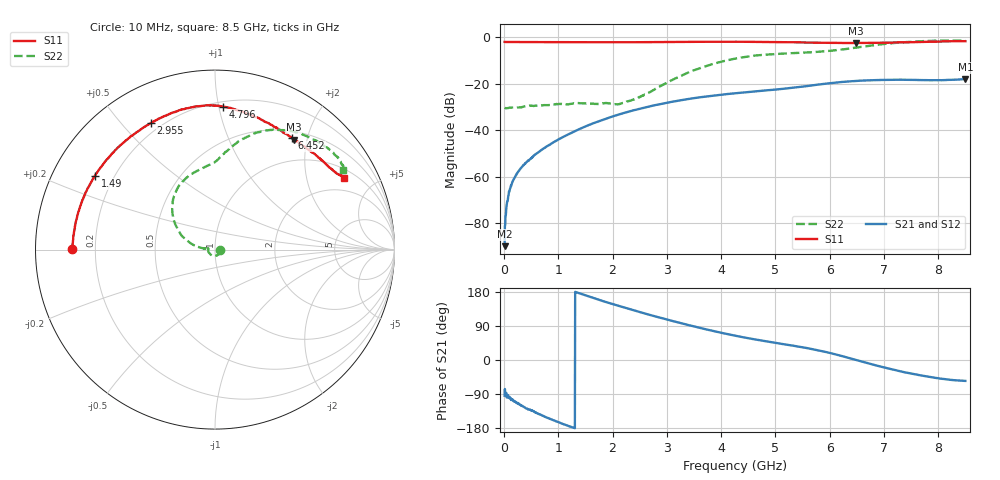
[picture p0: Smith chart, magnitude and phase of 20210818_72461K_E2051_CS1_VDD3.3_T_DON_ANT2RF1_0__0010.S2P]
!Agilent Technologies,E5071C,MY46417908,A.11.23
!Date: Wed Aug 18 14:23:20 2021
!Data & Calibration Information:
!Freq	S11:SOLT2(ON)	S21:SOLT2(ON)	S12:SOLT2(ON)	S22:SOLT2(ON)
!PortZ  Port1:50+j0  Port2:50+j0
!Above PortZ is port z conversion or system Z0 setting when saving the data.
!When reading, reference impedance value at option line is always used.
# Hz S dB R 50
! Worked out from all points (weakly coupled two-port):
!   1601 points, 10 MHz to 8.5 GHz, reference 50 ohm
!   highest |S21| = -17.98 dB at 8.5 GHz (marker M1); lowest = -89.8 dB at 10 MHz (marker M2)
!   lowest |S11| = -2.5 dB at 6.489 GHz (marker M3), VSWR 7.12, Z = 31.3 + j88.8 ohm
!   |S11| at or under -10 dB: nowhere
!   |S22| runs from -30.5 to -1.3 dB; largest |S21 - S12| = 0.00057
!   S11 on the Smith chart (normalised r, x): 10 MHz: 0.11, +0.00; 1.49 GHz: 0.13, +0.28; 2.955 GHz: 0.16, +0.60; 4.796 GHz: 0.24, +1.03; 6.452 GHz: 0.61, +1.75; 8.5 GHz: 1.34, +3.36
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1e7  -1.97 179.7  -89.78 -94.3  -86.23 -101.5  -30.29 -2.4
8.42875e7  -2.00 178.2  -67.82 -99.3  -67.36 -96.3  -30.30 -10.3
1.320438e8  -2.01 177.2  -63.86 -105.7  -63.77 -103.6  -30.22 -15.0
2.116375e8  -2.03 175.5  -59.63 -110.5  -59.69 -110.5  -30.17 -23.3
3.230688e8  -2.03 173.1  -55.81 -120.7  -55.80 -121.2  -30.01 -40.6
7.422625e8  -2.06 164.3  -47.60 -149.1  -47.62 -149.0  -29.16 -93.1
1.426769e9  -2.09 149.8  -39.04 174.0  -39.05 174.1  -28.37 -164.7
1.490444e9  -2.10 148.4  -38.41 171.0  -38.42 171.1  -28.43 -169.8
2.127194e9  -2.11 134.4  -33.09 142.2  -33.09 142.1  -28.71 168.2
2.466794e9  -2.10 127.1  -30.91 127.9  -30.91 127.8  -25.95 172.7
2.843538e9  -2.06 119.1  -28.88 112.8  -28.88 112.7  -21.41 172.0
2.954969e9  -2.04 116.8  -28.35 108.8  -28.35 108.8  -20.10 170.6
3.496206e9  -1.96 106.7  -26.17 88.7  -26.16 88.7  -14.18 158.1
4.255e9  -1.89 94.6  -24.06 64.2  -24.07 64.2  -9.19 132.9
4.796238e9  -1.97 86.8  -22.90 50.1  -22.90 50.2  -7.51 114.6
5.671769e9  -2.26 71.6  -20.68 29.1  -20.68 29.2  -6.40 91.9
6.451788e9  -2.44 55.3  -18.81 1.4  -18.83 1.3  -4.52 79.6
6.488931e9  -2.46 54.4  -18.77 -0.1  -18.79 -0.1  -4.42 78.9
7.088538e9  -2.25 42.4  -18.26 -22.6  -18.29 -22.8  -2.65 64.9
7.486506e9  -2.12 35.8  -18.30 -35.3  -18.30 -35.4  -1.94 54.2
7.937538e9  -1.82 30.9  -18.41 -46.9  -18.39 -46.9  -1.45 41.6
8.5e9  -1.67 29.1  -17.98 -55.2  -18.00 -55.4  -1.51 31.6
